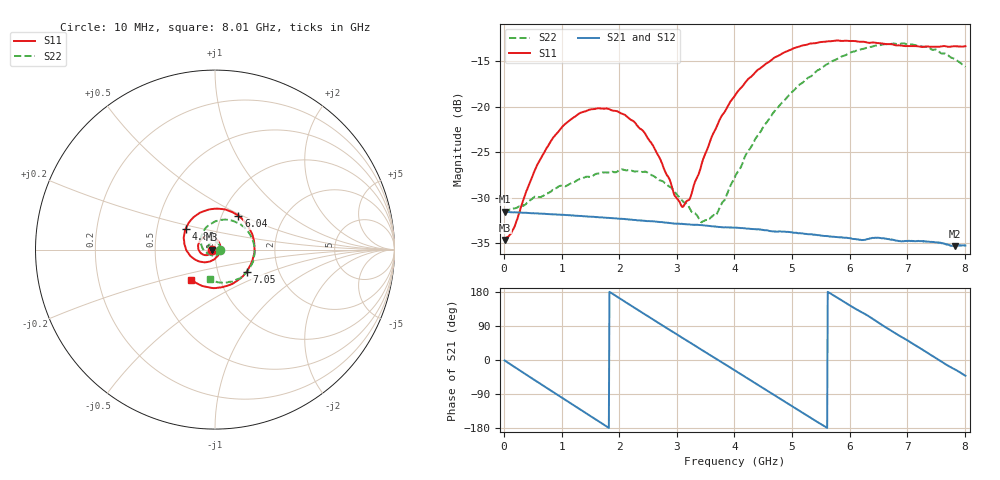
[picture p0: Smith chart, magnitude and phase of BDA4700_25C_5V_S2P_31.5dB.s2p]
!Agilent Technologies,E5071B,MY42404982,A.09.10
!Date: Mon Oct 20 13:42:30 2025
!Data & Calibration Information:
!Freq	S11:SOLT2(ON)	S21:SOLT2(ON)	S12:SOLT2(ON)	S22:SOLT2(ON)
# Hz S RI R 50
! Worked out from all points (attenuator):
!   801 points, 10 MHz to 8.01 GHz, reference 50 ohm
!   highest |S21| = -31.56 dB at 20 MHz (marker M1); lowest = -35.3 dB at 7.83 GHz (marker M2)
!   lowest |S11| = -34.7 dB at 10 MHz (marker M3), VSWR 1.04, Z = 48.2 - j0.094 ohm
!   |S11| at or under -10 dB: start of sweep to end of sweep
!   |S22| runs from -32.7 to -13.0 dB; largest |S21 - S12| = 0.00023
!   S11 on the Smith chart (normalised r, x): 10 MHz: 0.96, -0.00; 4.89 GHz: 0.70, +0.17; 6.04 GHz: 1.20, +0.48; 7.05 GHz: 1.37, -0.36; 8.01 GHz: 0.73, -0.26
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1e7  -0.0184 -0.000975  0.0264 -0.000582  0.0265 -0.000598  0.0263 -0.000816
2e7  -0.0187 -0.00152  0.0264 -0.000997  0.0264 -0.00103  0.0262 -0.00111
1.6e8  -0.0191 -0.0091  0.0252 -0.00731  0.0252 -0.00734  0.0264 -0.00758
5.4e8  -0.0354 -0.0282  0.0152 -0.0209  0.0152 -0.021  0.0157 -0.0278
7.8e8  -0.0535 -0.031  0.00554 -0.025  0.00558 -0.0251  0.000393 -0.0336
1.35e9  -0.093 0.00343  -0.0172 -0.0182  -0.0172 -0.0182  -0.0361 -0.0179
2.09e9  -0.0537 0.0725  -0.0218 0.0103  -0.0218 0.0103  -0.0294 0.0338
2.68e9  0.0152 0.0515  -0.00323 0.023  -0.00324 0.023  0.0126 0.0376
2.97e9  0.029 0.0137  0.00762 0.0214  0.00758 0.0214  0.0255 0.0218
3.12e9  0.0273 -0.00796  0.0125 0.0188  0.0125 0.0188  0.0281 0.00996
3.24e9  0.0208 -0.0243  0.0158 0.0159  0.0159 0.0159  0.027 0.00137
3.54e9  -0.0117 -0.0584  0.0212 0.00627  0.0212 0.00619  0.0131 -0.02
3.7e9  -0.0386 -0.0682  0.0218 0.00052  0.0219 0.000475  -0.00051 -0.0259
4.01e9  -0.0966 -0.0625  0.0191 -0.0101  0.0191 -0.0101  -0.032 -0.0257
4.89e9  -0.1641 0.1143  -0.00745 -0.0191  -0.00738 -0.0192  -0.0736 0.082
5.35e9  -0.0777 0.2082  -0.018 -0.00841  -0.0179 -0.00845  -0.0155 0.1474
6.04e9  0.1309 0.1882  -0.0145 0.0119  -0.0146 0.0119  0.139 0.1432
6.68e9  0.2202 -0.00183  0.0029 0.0184  0.00295 0.0185  0.2197 0.000579
7.05e9  0.176 -0.1233  0.0124 0.0135  0.0124 0.0134  0.1967 -0.0982
7.46e9  0.0564 -0.2055  0.0178 0.00268  0.0178 0.00263  0.1112 -0.1722
7.83e9  -0.0755 -0.2012  0.0155 -0.00719  0.0155 -0.0073  0.0139 -0.1818
8.01e9  -0.1317 -0.1692  0.0129 -0.0114  0.013 -0.0114  -0.03 -0.1623
